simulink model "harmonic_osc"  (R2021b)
settings: Solver=ode1  StartTime=0.0  StopTime=10  FixedStep=1e-4  RelTol=1e-3
undefined symbols (not defined in the file or in its folder): ca, cr, GM, Kr, M1, M2
libraries: fl_lib x14, nesl_utility x5, simulink x1

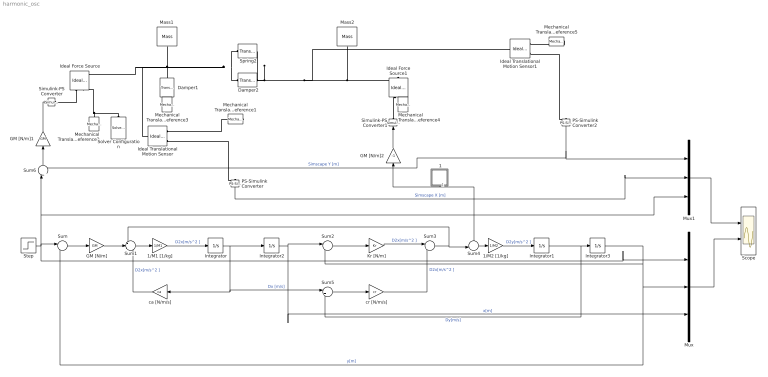
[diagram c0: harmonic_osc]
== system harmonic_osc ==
  " 1" : Subsystem  mask(Forze Esterne [ N]){FRC0=0, FRC=10, FRCt=3, FRR=1*0, FRR0=0, FRRt=4, FRA=0, FRSt=0, FRF=0}
      mask prompts: FRC0 "Valore iniziale FR (N):"; FRC "Forza finale FRC (N):"; FRCt "Istante applicazione FRC (s):"; FRR "Pendenza rampa FR (N/s):"; FRR0 "Valore iniziale rampa FR (N):"; FRRt "Istante applicazione FRR (s):"; FRA "Ampiezza carico sinusoidale FRA (N):"; FRSt "Istante applicazione FRA (s):"; FRF "Frequenza FRA (Hz):"
      mask help: Forza Aerodinamica agente sulla superficie mobile mossa dal martinetto:
  " Damper1" : fl_lib/Mechanical/Translational Elements/Translational Damper  D=20 N/(m/s)  v_specify=off  v_priority=None  v=0 m/s  v_nominal_specify=off  v_nominal_unit=m/s  v_nominal_value=1  f_specify=off  f_priority=None  f=0 N  f_nominal_specify=off  f_nominal_unit=N  f_nominal_value=1
  " Damper2" : fl_lib/Mechanical/Translational Elements/Translational Damper  D=5 N/(m/s)  v_specify=off  v_priority=None  v=0 m/s  v_nominal_specify=off  v_nominal_unit=m/s  v_nominal_value=1  f_specify=off  f_priority=None  f=0 N  f_nominal_specify=off  f_nominal_unit=N  f_nominal_value=1
  " Spring2" : fl_lib/Mechanical/Translational Elements/Translational Spring  spr_rate=1000 N/m  v_specify=off  v_priority=None  v=0 m/s  v_nominal_specify=off  v_nominal_unit=m/s  v_nominal_value=1  f_specify=off  f_priority=None  f=0 N  f_nominal_specify=off  f_nominal_unit=N  f_nominal_value=1  x_specify=off  x_priority=High  x=0 m  x_nominal_specify=off  x_nominal_unit=m  x_nominal_value=1
  1/M1 [1/kg] : Gain  Gain=1/M1
  1/M2 [1/kg] : Gain  Gain=1/M2
  GM [N/m] : Gain  Gain=GM
  GM [N/m]1 : Gain  Gain=GM
  GM [N/m]2 : Gain  Gain=-1
  Ideal Force Source : fl_lib/Mechanical/Mechanical Sources/Ideal Force Source
  Ideal Force Source1 : fl_lib/Mechanical/Mechanical Sources/Ideal Force Source
  Ideal Translational Motion Sensor : fl_lib/Mechanical/Mechanical Sensors/Ideal Translational Motion Sensor  offset=0 m
  Ideal Translational Motion Sensor1 : fl_lib/Mechanical/Mechanical Sensors/Ideal Translational Motion Sensor  offset=0 m
  Integrator{,1..3} (4 alike) : Integrator
  Kr [N/m] : Gain  Gain=Kr
  "Mass1 " : fl_lib/Mechanical/Translational Elements/Mass  mass=1 kg  num_ports=foundation.enum.numPorts2.one  v_specify=off  v_priority=High  v=0 m/s  v_nominal_specify=off  v_nominal_unit=m/s  v_nominal_value=1  f_specify=off  f_priority=None  f=0 N  f_nominal_specify=off  f_nominal_unit=N  f_nominal_value=1
  Mass2 : fl_lib/Mechanical/Translational Elements/Mass  mass=1 kg  num_ports=foundation.enum.numPorts2.one  v_specify=off  v_priority=High  v=0 m/s  v_nominal_specify=off  v_nominal_unit=m/s  v_nominal_value=1  f_specify=off  f_priority=None  f=0 N  f_nominal_specify=off  f_nominal_unit=N  f_nominal_value=1
  Mechanical Translational Reference{1..5} (5 alike) : fl_lib/Mechanical/Translational Elements/Mechanical Translational Reference
  Mux : Mux  Inputs=3
  Mux1 : Mux  Inputs=3
  PS-Simulink Converter : nesl_utility/PS-Simulink Converter  PhysicalDomain=network_engine_domain  SubClassName=ps_output  LeftPortType=input  RightPortType=output  PseudoPeriodic=off  Frequencies=[]  Unit=inherit  AffineConversion=off
  PS-Simulink Converter2 : nesl_utility/PS-Simulink Converter  PhysicalDomain=network_engine_domain  SubClassName=ps_output  LeftPortType=input  RightPortType=output  PseudoPeriodic=off  Frequencies=[]  Unit=inherit  AffineConversion=off
  Scope : Scope  NumInputPorts=2
  Simulink-PS Converter : nesl_utility/Simulink-PS Converter  PhysicalDomain=network_engine_domain  SubClassName=ps_input  LeftPortType=input  RightPortType=output  PseudoPeriodic=off  Frequencies=[]  NoiseDistribution=none  NoiseParameters=[]  Unit=1  AffineConversion=off  FilteringAndDerivatives=provide  SimscapeFilterOrder=1  InputFilterTimeConstant=0.001  UdotUserProvided=0
  Simulink-PS Converter1 : nesl_utility/Simulink-PS Converter  PhysicalDomain=network_engine_domain  SubClassName=ps_input  LeftPortType=input  RightPortType=output  PseudoPeriodic=off  Frequencies=[]  NoiseDistribution=none  NoiseParameters=[]  Unit=1  AffineConversion=off  FilteringAndDerivatives=provide  SimscapeFilterOrder=1  InputFilterTimeConstant=0.001  UdotUserProvided=0
  Solver Configuration : nesl_utility/Solver Configuration  PhysicalDomain=network_engine_domain  SubClassName=solver  LeftPortType=input  RightPortType=generic  Tones=[]  Harmonics=[]  SimulateNoise=off  Profile=off  UseLocalSampling=off  EnableSwitchedLinearOptims=on  FrequencyDomain=off  UseCCode=off  RelTol=0.001  AbsTol=1e-06  MinStep=1e-09  ToWorkspace=off  RevertToSquareIcSolve=off  NumHomotopyIterations=100  PhasorMode=off  PhasorModeNumHarmonics=1  DoDC=off  ResidualTolerance=1e-2  UseLocalSolver=off  LocalSolverChoice=NE_BACKWARD_EULER_ADVANCER  LocalSolverSampleTime=0.001  DoFixedCost=off  MaxNonlinIter=3  MaxModeIter=2  ComputeImpulses=off  ImpulseIterations=2  LinearAlgebra=auto  EquationFormulation=NE_TIME_EF  DelaysMemoryBudget=1024  AutomaticFiltering=on  FilteringTimeConstant=0.001  PartitionStorageMethod=AS_NEEDED  PartitionMemoryBudget=1024  PartitionMethod=ROBUST
  Step : Step  SampleTime=0
  Sum{,2,5..6} (4 alike) : Sum  Inputs=|+-
  Sum1 : Sum  Inputs=-+-
  Sum3 : Sum  Inputs=|++
  Sum4 : Sum  Inputs=-+|
  ca [N/m/s] : Gain  Gain=ca
  cr [N/m/s] : Gain  Gain=cr
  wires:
  Sum/1 -> GM [N/m]/1
  Step/1 -> Mux/1, Sum/1, Mux1/3, Sum6/1
  GM [N/m]/1 -> Sum1/2
  Sum1/1 -> 1/M1 [1/kg]/1
  1/M1 [1/kg]/1 -> Integrator/1  "D2x[m/s^2 ]"
  Integrator/1 -> Sum5/1, ca [N/m/s]/1, Integrator2/1  "Dx [m/s]"
  Sum2/1 -> Kr [N/m]/1
  Integrator2/1 -> Mux/3, Sum2/1  "x[m]"
  Kr [N/m]/1 -> Sum3/1  "D2x[m/s^2 ]"
  Sum3/1 -> Sum1/1, Sum4/2
  cr [N/m/s]/1 -> Sum3/2  "D2x[m/s^2 ]"
  Sum5/1 -> cr [N/m/s]/1
  ca [N/m/s]/1 -> Sum1/3  "D2x[m/s^2 ]"
  Sum4/1 -> 1/M2 [1/kg]/1
  1/M2 [1/kg]/1 -> Integrator1/1  "D2y[m/s^2 ]"
  Integrator1/1 -> Sum5/2, Integrator3/1  "Dy[m/s]"
  Integrator3/1 -> Sum2/2, Sum/2, Mux/2  "y[m]"
  " 1"/1(FR) -> Sum4/1, GM [N/m]2/1
  GM [N/m]2/1 -> Simulink-PS Converter1/1
  GM [N/m]1/1 -> Simulink-PS Converter/1
  Sum6/1 -> GM [N/m]1/1
  PS-Simulink Converter/1 -> Mux1/2  "Simscape X [m]"
  PS-Simulink Converter2/1 -> Sum6/2, Mux1/1  "Simscape Y [m]"
  Mux1/1 -> Scope/1
  Mux/1 -> Scope/2
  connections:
  Solver Configuration/RConn1 -- Ideal Force Source/RConn2 -- Mechanical Translational Reference2/LConn1
  " Damper2"/RConn1 -- Ideal Translational Motion Sensor1/LConn1 -- Mass2/LConn1 -- Ideal Force Source1/LConn1 -- " Spring2"/RConn1
  Mechanical Translational Reference1/LConn1 -- Ideal Translational Motion Sensor/RConn1
  Ideal Translational Motion Sensor/RConn3 -- PS-Simulink Converter/LConn1
  Ideal Force Source/RConn1 -- Simulink-PS Converter/RConn1
  " Damper2"/LConn1 -- Ideal Translational Motion Sensor/LConn1 -- Ideal Force Source/LConn1 -- " Damper1"/LConn1 -- "Mass1 "/LConn1 -- " Spring2"/LConn1
  Mechanical Translational Reference3/LConn1 -- " Damper1"/RConn1
  Simulink-PS Converter1/RConn1 -- Ideal Force Source1/RConn1
  Mechanical Translational Reference4/LConn1 -- Ideal Force Source1/RConn2
  Mechanical Translational Reference5/LConn1 -- Ideal Translational Motion Sensor1/RConn1
  Ideal Translational Motion Sensor1/RConn3 -- PS-Simulink Converter2/LConn1

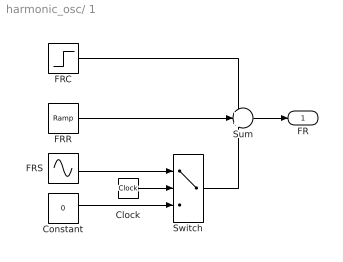
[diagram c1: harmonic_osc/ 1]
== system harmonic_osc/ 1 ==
  Clock : Clock
  Constant : Constant  Value=0
  FRC : Step  Time=FRCt  Before=FRC0  After=FRC  SampleTime=0
  FRR : simulink/Sources/Ramp  slope=FRR  start=FRRt  InitialOutput=FRR0
  FRS : Sin  Amplitude=FRA  Frequency=2*pi*FRF  Phase=-2*pi*FRF*FRSt  SampleTime=0
  Sum : Sum  Inputs=+++
  Switch : Switch  Threshold=FRSt
  FR : Outport
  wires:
  FRC/1 -> Sum/1
  FRR/1 -> Sum/2
  Sum/1 -> FR/1
  Switch/1 -> Sum/3
  Constant/1 -> Switch/3
  Clock/1 -> Switch/2
  FRS/1 -> Switch/1
